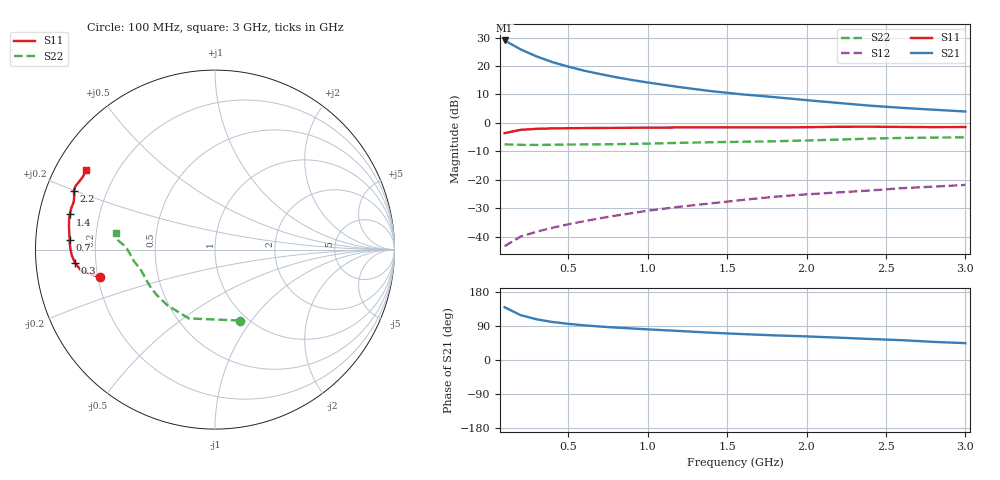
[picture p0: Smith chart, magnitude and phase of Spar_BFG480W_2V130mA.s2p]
! Filename: 2130BFG480.001
! Title: BFG480W
! Bias: Vce=2V; Ic=130mA
! Company: NXP Semiconductors NL
! User: Quality&Reliability T&D
! Measure time: 10 Nov 1999 / 11:55:36
#  MHz  S  MA  R 50
! Freq  S11  S21  S12  S22  :
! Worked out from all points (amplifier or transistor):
!   20 points, 100 MHz to 3 GHz, reference 50 ohm
!   highest |S21| = 29.0 dB at 100 MHz (marker M1)
!   |S21| within 3 dB of that: start of sweep to 196.2 MHz
!   unconditionally stable (mu >= 1): start of sweep to end of sweep
!   at 400 MHz: K = 1.15, MAG = 26.8 dB, |S12| = -36.9 dB
!   at 1.2 GHz: K = 1.27, MAG = 17.9 dB, |S12| = -29.5 dB
!   at 3 GHz: K = 1.27, MAG = 9.8 dB, |S12| = -21.8 dB
!   S11 on the Smith chart (normalised r, x): 100 MHz: 0.21, -0.11; 300 MHz: 0.12, -0.05; 700 MHz: 0.10, +0.03; 1.4 GHz: 0.09, +0.12; 2.2 GHz: 0.08, +0.20; 3 GHz: 0.09, +0.28
100  0.6586 -166.5  28.07 139.2  0.006784 61.7  0.4184 -70.9
200  0.7527 -170.8  19.6 118.5  0.009988 56.1  0.4101 -110.8
300  0.7842 -174.7  14.76 107.5  0.01214 57.4  0.4086 -130.8
400  0.7981 -177.6  11.7 100.5  0.01427 60.3  0.4113 -141.9
500  0.8046 -179.9  9.73 95.4  0.01642 63.1  0.415 -149.0
600  0.8094 178.0  8.263 91.5  0.01863 65.2  0.4174 -153.9
700  0.8118 176.2  7.213 88.3  0.02096 67.2  0.4194 -157.6
800  0.8146 174.5  6.355 85.6  0.02337 69.0  0.4219 -160.6
900  0.8185 172.9  5.667 83.2  0.02579 70.7  0.4256 -163.2
1000  0.8225 171.4  5.128 80.9  0.0285 71.3  0.431 -165.5
1200  0.8294 168.7  4.252 76.5  0.03345 72.7  0.4441 -169.1
1400  0.8326 166.4  3.604 72.0  0.03841 73.3  0.4564 -171.9
1600  0.8336 163.9  3.157 68.3  0.04413 73.7  0.4645 -174.4
1800  0.8305 161.4  2.825 65.0  0.05017 73.8  0.4741 -177.1
2000  0.8381 159.4  2.507 62.3  0.05532 74.2  0.4886 179.8
2200  0.8521 157.4  2.237 59.0  0.05976 74.1  0.5077 177.3
2400  0.8538 155.5  2.003 55.5  0.06462 73.4  0.528 175.7
2600  0.8468 153.5  1.834 52.3  0.07099 72.5  0.5421 174.5
2800  0.8403 151.1  1.7 47.8  0.07556 71.0  0.549 172.8
3000  0.8439 148.4  1.581 44.5  0.08096 70.1  0.5573 170.2
